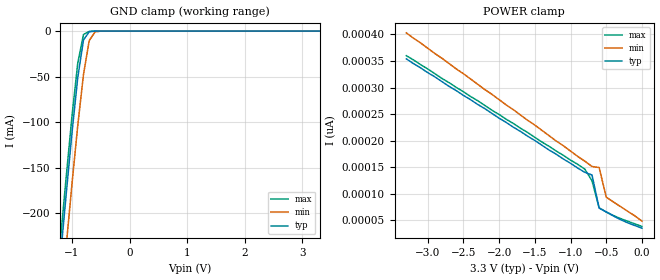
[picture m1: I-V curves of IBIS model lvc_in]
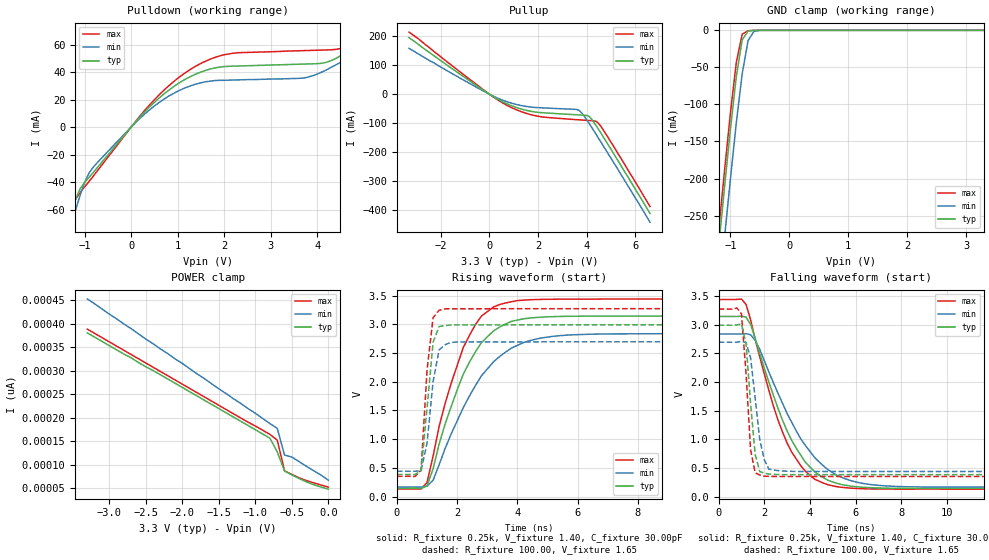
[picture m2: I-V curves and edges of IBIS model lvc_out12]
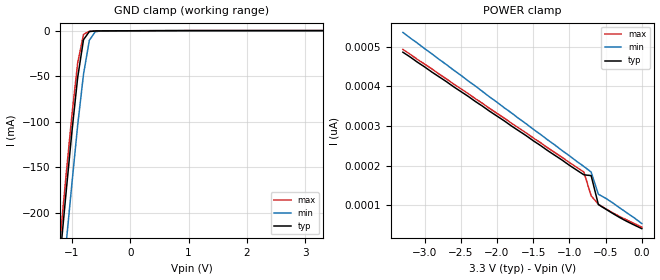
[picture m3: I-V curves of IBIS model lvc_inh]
| IBIS file 162244xh.ibs created by s2ibis2 version 1.1
| North Carolina State University Electronics Research Laboratory  1995
[IBIS ver]   2.1
[File name]   162244xh.ibs
[File Rev]   1.0
[Date]   03/01/99 rtk rtk
[Source]   Integrated Device Technology, Inc.
[Notes]   1.Temperatures: typ=25C, min=100C, max=0C 2.RRmp rates based
   on 50 ohm load.
[Disclaimer] Integrated Device Technology, Inc. ("IDT") hereby grants the
   user of this IBIS model a non-exclusive, nontransferable
   license to use this IBIS model under the following terms. The
   user is granted this license only to use the IBIS model and is
   not granted rights to sell, copy (except as needed to run the
   IBIS model), rent, lease or sub-license the IBIS model in
   whole or in part, or in modified form to anyone. The User may
   modify the IBIS model to suit its specific applications, but
   rights to derivative works and such modifications shall belong
   to IDT. This IBIS model is provided on an AS IS" basis and IDT
   makes absolutely no warranty with respect to the information
   contained herein. IDT DISCLAIMS AND CUSTOMER WAIVES ALL
   WARRANTIES, EXPRESS AND IMPLIED, INCLUDING WARRANTIES OF
   MERCHANTABILITY AND FITNESS FOR A PARTICULAR PURPOSE. THE
   ENTIRE RISK AS TO QUALITY AND PERFORMANCE IS WITH THE USER
   ACCORDINGLY, IN NO EVENT SHALL IDT BE LIABLE FOR ANY DIRECT OR
   INDIRECT DAMAGES, WHETHER IN CONTRACT OR TORT, INCLUDING ANY
   LOST PROFITS OR OTHER INCIDENTAL, CONSEQUENTIAL, EXEMPLARY, OR
   PUNITIVE DAMAGES ARISING OUT OF THE USE OR APPLICATION OF THE
   IBIS model. Further, IDT reserves the right to make changes
   without notice to any product herein to improve reliability,
   function, or design. IDT does not convey any license under
   patent rights or any other intellectual property rights,
   including those of third parties. IDT is not obligated to
   provide maintenance or support for the licensed IBIS model.
[Copyright]   Copyright 1997, Integrated Device Technology, Inc. all rights
   reserved
|   Component LVCH162244
[Component]   LVCH162244
[Manufacturer]   Integrated Device Technology
[Package]
| PA48
| variable   typ   min   max
R_pkg   6.50m   5.00m   10.00m
L_pkg   3.20nH   2.50nH   4.40nH
C_pkg   0.27pF   0.01pF   0.98pF
| PV48   typ   min   max
|R_pkg   6.5m   5.00m   10.00m
|L_pkg   4.75nH   3.82nH   6.72nH
|C_pkg   0.24pF   0.01pF   1.55pF
[Pin]  signal_name   model_name   R_pin   L_pin   C_pin
1   1OEB   lvc_in
2   1Y1   lvc_out12
3   1Y2   lvc_out12
4   GND   GND
5   1Y3   lvc_out12
6   1Y4   lvc_out12
7   VCC   POWER
8   2Y1   lvc_out12
9   2Y2   lvc_out12
10   GND   GND
11   2Y3   lvc_out12
12   2Y4   lvc_out12
13   3Y1   lvc_out12
14   3Y2   lvc_out12
15   GND   GND
16   3Y3   lvc_out12
17   3Y4   lvc_out12
18   VCC   POWER
19   4Y1   lvc_out12
20   4Y2   lvc_out12
21   GND   GND
22   4Y3   lvc_out12
23   4Y4   lvc_out12
24   4OEB   lvc_in
25   3OEB   lvc_in
26   4A4   lvc_inh
27   4A3   lvc_inh
28   GND   GND
29   4A2   lvc_inh
30   4A1   lvc_inh
31   VCC   POWER
32   3A4   lvc_inh
33   3A3   lvc_inh
34   GND   GND
35   3A2   lvc_inh
36   3A1   lvc_inh
37   2A4   lvc_inh
38   2A3   lvc_inh
39   GND   GND
40   2A2   lvc_inh
41   2A1   lvc_inh
42   VCC   POWER
43   1A4   lvc_inh
44   1A3   lvc_inh
45   GND   GND
46   1A2   lvc_inh
47   1A1   lvc_inh
48   2OEB   lvc_in
| Models and submodels in the file (3): lvc_in (Input), lvc_out12 (3-state), lvc_inh (Input)
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| in   in   dummy_model
| oe   oe
|   Model lvc_in
[Model]   lvc_in
Model_type   Input
Vinl =  0.800V
Vinh =  2.000V
C_comp   3.00pF   NA   NA
[Temperature Range]   25.00   100.00   0.000
[Voltage Range]   3.30V   3.00V   3.60V
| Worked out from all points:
|   GND clamp passes 1 mA (typ) near -0.70 V on its own axis
[GND_clamp]
| voltage   I(typ)   I(min)   I(max)
-3.3V     -1.806A    -1.858A    -1.789A
-1.2V     -248mA     -306mA     -229mA
-1.1V     -179mA     -236mA     -160mA
-1V       -112mA     -168mA     -93.56mA
-900mV    -51.39mA   -104mA     -35.36mA
-800mV    -9.697mA   -47.7mA    -3.786mA
-700mV    -714uA     -10.4mA    -348uA
-600mV    -52.42uA   -951uA     -8.225uA
-500mV    -126nA     -30.48uA   -10.89nA
3.3V      34.69pA    75.27pA    23pA
[POWER_clamp]
| voltage   I(typ)   I(min)   I(max)
-3.3V     354pA      403pA      360pA
-800mV    140pA      161pA      146pA
-700mV    135pA      151pA      124pA
-600mV    72.75pA    149pA      72.79pA
-500mV    65.09pA    93.05pA    65.39pA
-300mV    50.77pA    75.27pA    52.78pA
0V        34.68pA    47.91pA    37.83pA
|   Model lvc_out12
[Model]   lvc_out12
Model_type   3-state
Polarity   Non-Inverting
Enable   Active-High
Vinl =  0.000V
Vinh =  2.000V
Vmeas =  1.500V
C_comp   3.00pF   NA   NA
[Temperature Range]   25.00   100.00   0.000
[Voltage Range]   3.30V   3.00V   3.60V
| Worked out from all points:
|   slope of the pulldown table from 0 to 0.495 V, typ, clamps not added: 27.7 ohm
|   slope of the pullup table from 0 to 0.495 V, typ, clamps not added: 20.6 ohm
|   GND clamp passes 1 mA (typ) near -0.70 V on its own axis
|   rising waveform, R_fixture 0.25k, V_fixture 1.40, C_fixture 30.00pF: 20-80 % time 1.31ns typ, 1.63ns min, 1.14ns max; typ from 0.143 V to 3.15 V
|   rising waveform, R_fixture 100.00, V_fixture 1.65: 20-80 % time 278ps typ, 304ps min, 252ps max; typ from 0.384 V to 2.99 V
|   falling waveform, R_fixture 0.25k, V_fixture 1.40, C_fixture 30.00pF: 20-80 % time 1.8ns typ, 2.1ns min, 1.6ns max; typ from 3.15 V to 0.143 V
|   falling waveform, R_fixture 100.00, V_fixture 1.65: 20-80 % time 324ps typ, 409ps min, 285ps max; typ from 2.99 V to 0.384 V
[Pulldown]
| voltage   I(typ)   I(min)   I(max)
-3.3V     -319mA     -329mA     -316mA
-1.4V     -75mA      -84.8mA    -72.4mA
-1.3V     -63.5mA    -72.8mA    -61.6mA
-900mV    -36.4mA    -33.1mA    -39.4mA
47.68nV   1.93nA     1.67nA     2.11nA
900mV     29.1mA     24.3mA     32.7mA
1.7V      42.3mA     33.5mA     49.5mA
3.8V      46mA       36.4mA     55.8mA
4.5V      51.9mA     47.1mA     57.2mA
5.4V      72.8mA     65.6mA     76mA
5.8V      83.6mA     74.6mA     87.3mA
6.6V      106mA      93.6mA     112mA
[Pullup]
| voltage   I(typ)   I(min)   I(max)
-3.3V     195mA      158mA      214mA
-300mV    16.6mA     13.3mA     18.8mA
700mV     -32.2mA    -25.2mA    -37.1mA
1.3V      -50.8mA    -38.9mA    -59.8mA
1.9V      -61.5mA    -45.8mA    -74.3mA
3.5V      -70.5mA    -52mA      -87.3mA
3.7V      -71.4mA    -56.7mA    -88.4mA
4.1V      -76.8mA    -101mA     -90.7mA
4.4V      -110mA     -140mA     -94mA
4.5V      -123mA     -154mA     -102mA
5.1V      -204mA     -235mA     -179mA
6.6V      -411mA     -441mA     -387mA
[GND_clamp]
| voltage   I(typ)   I(min)   I(max)
-3.3V     -2.114A    -2.176A    -2.094A
-1.2V     -293mA     -361mA     -271mA
-1.1V     -212mA     -280mA     -190mA
-1V       -134mA     -201mA     -112mA
-900mV    -62.73mA   -125mA     -43.63mA
-800mV    -12.84mA   -58.84mA   -5.255mA
-700mV    -1.029mA   -13.85mA   -500uA
-600mV    -75.02uA   -1.372mA   -11.67uA
-500mV    -184nA     -44.39uA   -15.73nA
3.3V      47.54pA    96.2pA     38.25pA
[POWER_clamp]
| voltage   I(typ)   I(min)   I(max)
-3.3V     380pA      452pA      388pA
-800mV    156pA      187pA      164pA
-700mV    127pA      177pA      152pA
-600mV    85.98pA    120pA      86.78pA
-500mV    77.97pA    116pA      78.98pA
-300mV    62.97pA    96.2pA     65.7pA
0V        47.54pA    66.68pA    51.85pA
[Ramp]
| variable   typ   min   max
dV/dt_r   1.26/0.25n   1.02/0.31n   1.46/0.27n
dV/dt_f   1.06/0.42n   0.85/0.53n   1.24/0.40n
R_load = 50.00
[Rising Waveform]
R_fixture = 0.25k
V_fixture = 1.40
C_fixture = 30.00pF
R_dut = 7.00m
L_dut = 3.30nH
C_dut = 0.29pF
| time   V(typ)   V(min)   V(max)
0s        143mV      165mV      131mV
1ns       187mV      180mV      248mV
1.2ns     483mV      283mV      704mV
1.6ns     1.266V     838mV      1.622V
2.2ns     2.129V     1.546V     2.594V
2.8ns     2.679V     2.101V     3.141V
3.4ns     2.95V      2.436V     3.344V
4.4ns     3.109V     2.715V     3.428V
5.8ns     3.14V      2.817V     3.439V
19.8ns    3.145V     2.838V     3.44V
[Rising Waveform]
R_fixture = 100.00
V_fixture = 1.65
R_dut = 7.00m
L_dut = 3.30nH
C_dut = 0.29pF
| time   V(typ)   V(min)   V(max)
0s        384mV      440mV      352mV
600ps     383mV      439mV      348mV
800ps     446mV      450mV      461mV
1ns       1.541V     932mV      2.205V
1.2ns     2.69V      2.005V     3.116V
1.4ns     2.961V     2.556V     3.245V
1.6ns     2.978V     2.645V     3.27V
1.8ns     2.988V     2.686V     3.271V
2ns       2.99V      2.691V     3.27V
19.8ns    2.991V     2.695V     3.273V
[Falling Waveform]
R_fixture = 0.25k
V_fixture = 1.40
C_fixture = 30.00pF
R_dut = 7.00m
L_dut = 3.30nH
C_dut = 0.29pF
| time   V(typ)   V(min)   V(max)
0s        3.145V     2.838V     3.44V
1.2ns     3.133V     2.844V     3.355V
1.6ns     2.763V     2.727V     2.746V
2.4ns     1.765V     1.985V     1.578V
3ns       1.144V     1.449V     932mV
3.8ns     598mV      891mV      441mV
4.6ns     329mV      532mV      234mV
5.8ns     182mV      277mV      148mV
7.4ns     148mV      186mV      133mV
19.8ns    143mV      165mV      131mV
[Falling Waveform]
R_fixture = 100.00
V_fixture = 1.65
R_dut = 7.00m
L_dut = 3.30nH
C_dut = 0.29pF
| time   V(typ)   V(min)   V(max)
0s        2.991V     2.695V     3.273V
1ns       3.011V     2.71V      3.19V
1.2ns     2.664V     2.688V     2.151V
1.4ns     1.621V     2.419V     815mV
1.6ns     735mV      1.719V     419mV
1.8ns     438mV      994mV      378mV
2ns       412mV      643mV      357mV
2.2ns     394mV      480mV      355mV
2.8ns     384mV      447mV      352mV
19.8ns    384mV      440mV      352mV
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|   Model lvc_inh
[Model]   lvc_inh
Model_type   Input
Vinl =  0.800V
Vinh =  2.000V
C_comp   3.00pF   NA   NA
[Temperature Range]   25.00   100.00   0.000
[Voltage Range]   3.30V   3.00V   3.60V
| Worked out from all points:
|   GND clamp passes 1 mA (typ) near -0.70 V on its own axis
[GND_clamp]
| voltage   I(typ)   I(min)   I(max)
-3.3V     -1.806A    -1.858A    -1.789A
-1.2V     -248mA     -306mA     -229mA
-1.1V     -179mA     -236mA     -160mA
-1V       -112mA     -169mA     -93.63mA
-900mV    -51.47mA   -104mA     -35.47mA
-800mV    -9.82mA    -47.77mA   -3.967mA
-700mV    -887uA     -10.48mA   -557uA
-600mV    -219uA     -1.066mA   -201uA
-500mV    -136uA     -141uA     -155uA
3.3V      163uA      116uA      211uA
[POWER_clamp]
| voltage   I(typ)   I(min)   I(max)
-3.3V     486pA      536pA      493pA
-800mV    177pA      198pA      184pA
-700mV    175pA      184pA      124pA
-600mV    102pA      128pA      103pA
-500mV    90.69pA    118pA      91.59pA
-300mV    68.77pA    93pA       71.38pA
0V        41.28pA    54.13pA    45.03pA
